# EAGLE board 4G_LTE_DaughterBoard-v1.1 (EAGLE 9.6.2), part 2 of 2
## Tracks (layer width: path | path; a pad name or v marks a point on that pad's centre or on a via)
$$$29
  Bottom 0.203: U11.8 R17.1
  Bottom 0.305: R17.1 R18.2
+BAT  (via drill 0.35)
  Top 0.508: U3.3 19.02,104.75 | 22.34,99.86 22.29,99.91 v22.32,99.94 | v18.14,103.86 18.24,103.96
  Top 0.61: 19.02,104.75 C26.1 18.24,103.96 | BATTERY.2 22.34,99.86
  Bottom 0.61: v22.32,99.94 20.94,99.94 18.14,102.74 v18.14,103.86
  pour Top (isolate 0.254, no thermals): 28.27,101.11 35.49,101.11 36.05,100.55 36.05,98.89 35.74,98.58 33.85,98.58 33.47,98.96 28.27,98.96
AGND  (via drill 0.3)
  Top 0.406: J3.2 36.16,114.78 v35.95,114.99
  Bottom 0.203: U7.7 41.78,105.72 41.96,105.54 41.96,104.75 42.38,104.33 42.38,103.64 42.43,103.59 42.43,102.87 C51.2 | U7.18 36.73,105.72 36.38,105.36 36.38,105.16 36.18,104.96 35.78,104.96 | C57.1 C56.1 | C56.1
  Bottom 0.305: v45.19,105.6 45.19,105.96 45.28,106.05 45.28,107.82 v45.1,108
  other vias: 44.92,102.31 34.37,105.21 34.67,103.11 30.45,110.39 25.85,107.69 40.75,101.89 40.85,98.49 44.25,98.69
  pour Bottom (isolate 0.254, rank 2, no thermals): 22.78,96.56 22.78,115.76 41.18,115.76 41.38,115.56 41.38,113.76 41.48,113.36 41.58,112.76 41.78,112.36 41.98,112.06 44.93,111.59 45.58,111.26 45.58,99.86 45.41,96.56
  pour Route2 (isolate 0.254): 22.78,115.76 22.78,96.56 45.38,96.56 45.38,111.46 45.08,111.76 43.38,111.76 41.48,113.66 41.48,115.76
ANT_DIV
  Top 0.293: U1.35 30.77,45.7 arc45 31.13,44.82 arc45 32.48,44.26 35.82,44.26 arc90 37.97,46.41 C70.2 38.98,56.62 L3.1
ANT_GNSS
  Top 0.293: U1.47 C74.2 38.97,62.59 C83.2
ANT_MAIN
  Top 0.293: U1.49 C68.2 38.97,68.29 L2.1
AP_READY_EC25  (via drill 0.3, 0.41)
  Top 0.203: U1.2 v2.34,73.5 v2.33,73.49
  Route2 0.203: v3.5,22.12 3.5,21.95 9.69,15.76 13.4,15.76 14.38,14.78 v14.38,12.46
  Bottom 0.203: Q6.3 14.28,11.66 R44.2 v14.38,12.46 | v2.33,73.49 3.04,73.49 5.97,70.56 5.97,61.5 5.15,60.67 5.15,52.04 6.78,50.41 6.78,43.19 2.22,38.63 2.22,23.79 3.48,22.53 3.48,22.14 v3.5,22.12
BT_EN  (via drill 0.3)
  Top 0.203: U1.139 6.52,53.09 v5.81,52.38 | v22,36.75 22,34.82 22.3,34.52 U2.10 27.35,34.52 C19.1
  Route2 0.203: v22,36.75 22,36.67 21.56,36.23 9.79,36.23 9.49,35.93 9.49,35.92 9.27,35.7 6.45,35.7 6.21,35.94 6.21,46.59 5.56,47.24 v5.56,47.87
  Route15 0.203: v5.81,52.38 5.81,47.93 5.75,47.87 v5.56,47.87
CODEC_PCM_CLK  (via drill 0.3)
  Top 0.203: R38.1 20.33,44.8 v20.33,42.67
  Route2 0.203: v42.68,89.48 42.68,88.43 39.79,85.54 39.79,79.12 37.21,76.54 32.73,76.54 28.85,72.66 28.85,55.45 23.48,50.08 23.48,45.09 21.06,42.67 v20.33,42.67
  Route15 0.203: v33.76,110.24 33.95,110.05 34.52,110.05 36.33,108.24 38.66,108.24 39.18,107.73 39.18,95.36 42.38,92.16 42.38,89.78 v42.68,89.48
  Bottom 0.152: v33.76,110.24 33.78,110.22 33.78,110.06
  Bottom 0.203: R66.2 34.57,110.06 33.78,110.06
CODEC_PCM_IN  (via drill 0.3)
  Top 0.203: R32.1 16.42,44.79 v16.42,42.9
  Route2 0.203: v41,91.46 40.4,90.86 40.4,87.67 38.72,85.99 38.72,79.56 36.77,77.61 32.28,77.61 27.78,73.1 27.78,55.89 22.41,50.52 22.41,45.58 21.04,44.21 17.73,44.21 v16.42,42.9
  Route15 0.203: v32.55,106.14 32.56,106.13 36.02,106.13 38.11,104.04 38.11,94.35 v41,91.46
  Bottom 0.203: R69.2 34.65,107.32 33.65,106.32 32.72,106.32 v32.55,106.14 C53.2
CODEC_PCM_OUT  (via drill 0.3)
  Top 0.203: R34.1 17.73,44.8 v17.73,42.67
  Route2 0.203: v41.24,90.08 40.9,89.74 40.9,87.66 39.08,85.84 39.08,79.41 36.92,77.25 32.43,77.25 28.14,72.96 28.14,55.74 22.77,50.38 22.77,45.39 21.22,43.84 19.04,43.84 17.87,42.67 v17.73,42.67
  Route15 0.203: v32.77,109.63 33.12,109.28 33.12,108.86 33.95,108.03 34.62,108.03 38.47,104.18 38.47,95.04 41.67,91.85 41.67,90.51 v41.24,90.08
  Bottom 0.203: R68.2 33.87,108.12 33.77,108.22 33.77,108.43 C54.2 32.77,109.43 v32.77,109.63
CODEC_PCM_SYNC  (via drill 0.3)
  Top 0.203: R36.1 19.08,42.9 v19.03,42.85
  Route2 0.203: v41.69,88.89 41.69,87.95 39.43,85.69 39.43,79.26 37.06,76.9 32.58,76.9 28.49,72.81 28.49,55.59 23.12,50.23 23.12,45.24 21.36,43.47 19.65,43.47 v19.03,42.85
  Route15 0.203: v41.69,88.89 41.69,89.6 42.02,89.94 42.02,92.01 38.83,95.21 38.83,104.43 v34.28,108.98
  Bottom 0.203: R67.2 34.78,108.98 v34.28,108.98
CODEC_POWER_EN  (via drill 0.3, 0.35)
  Top 0.203: v15.15,81.45 15.11,81.45 14.45,82.11 14.45,88.43 14.88,88.86 15.93,88.86 16.38,89.31 Q10.1 | v26.08,7.92 7.02,7.92 v2.13,12.81
  Route15 0.203: v15.15,81.45 15.15,75.62 14.48,74.95 14.48,74.41 16.12,72.77 29.05,72.77 32.77,69.05 32.77,57.19 31.94,56.37 31.94,49.08 32.95,48.07 32.95,37.3 35.29,34.96 35.29,22.07 28.09,14.87 28.09,10.02 26.08,8.01 v26.08,7.92
  Bottom 0.203: WIPHONE_DAUGHTERBOARD-FOOTPRINT1.17 2.48,12.46 v2.13,12.81
COEX_UART_RX  (via drill 0.3)
  Top 0.203: U1.137 6.52,57.01 v5.9,56.39 | v22.45,29.02 v22.47,29 22.49,29.02 U2.5 27.4,29.02 R29.1
  Route2 0.203: v2.68,41.02 4.55,39.15 4.55,29.62 5.18,29 7.34,29 8.27,29 10.06,27.22 20.66,27.22 v22.45,29.02
  Route15 0.203: v5.9,56.39 3.77,54.26 3.77,49.64 1.58,47.45 1.58,42.12 v2.68,41.02
COEX_UART_TX  (via drill 0.3)
  Top 0.203: U1.138 6.52,55.05 v5.9,54.43 | v22.25,30.01 24.01,30.01 U2.6 27.42,30.12 R28.1
  Route2 0.203: v3.53,41.56 4.91,40.18 4.91,29.77 5.33,29.35 7.19,29.35 7.2,29.36 8.42,29.36 10.2,27.57 19.84,27.57 22.2,29.93 22.2,30.01 v22.25,30.01
  Route15 0.203: v5.9,54.43 4.13,52.67 4.13,49.51 1.99,47.37 1.99,43.1 v3.53,41.56
CTS_BT  (via drill 0.3)
  Top 0.203: U1.40 v33.31,53.5 | U2.8 25.87,32.32 26.15,32.6 v26.49,32.6
  Route2 0.203: v33.31,53.5 33.31,53.41 24.32,44.43 v24.32,39.83
  Bottom 0.203: v24.32,39.83 25.3,38.85 25.3,33.59 26.29,32.6 v26.49,32.6
DBG_RXD
  Top 0.203: U1.11 TP1.P$1
DBG_TXD
  Top 0.203: U1.12 2.15,57.4 TP2.P$1
DBG_TXD_FC20
  Top 0.203: U2.4 26.35,27.92 27.26,27.92 R30.1
DTR  (via drill 0.35)
  Route2 0.203: v7.35,8.64 7.35,7.84 v6.65,7.14
  Bottom 0.203: R86.1 R85.1 7.42,7.14 v6.65,7.14 | WIPHONE_DAUGHTERBOARD-FOOTPRINT1.20 7.35,8.54 v7.35,8.64
FC20_ANT
  Top 0.293: L4.1 8.09,25.86 C72.2 11.24,25.86 U2.30
GND  (via drill 0.3, 0.35, 0.41, 0.5)
  Top 0.203: C18.2 28.88,32.99 v28.99,33.1
  Top 0.229: U1.19 9.97,49.32 10.21,49.56 13.65,49.56 13.87,49.34 U1.22
  Top 0.305: D3.A 37.27,102.33 C90.1 | R58.2 16.83,84.02 17.95,84.02 v18.37,84.44 | v22.43,13.84 22.26,13.67 16.47,13.67 16.28,13.86 | 15.98,14.16 v15.98,16.9 | 16.28,13.86 15.98,14.16 | v16.28,13 16.28,13.86 | 15.98,14.16 15.66,13.84 v9.23,13.84 9.23,17.59 v9.59,17.95
  Top 0.406: U3.2 18.34,106.06 v18.3,106.1
  Top 0.508: C45.1 C44.1 17.34,86.56 U5.2 v20.88,86.56 | Q10.2 17.38,88.79 v17.1,88.51
  Route2 0.203: v2.55,16.44 2.55,13.32 2.79,13.08 2.79,9.9 6.87,5.82 v8.49,5.82
  Route15 0.305: v35.98,14.06 35.98,13.16 37.88,11.26 37.88,8.56 37.68,8.36 v37.48,8.36
  Bottom 0.203: C65.1 C66.1 | C53.1 32.5,104.56 v31.89,104.56 v31.88,104.56 | C52.1 34.35,111.08 v34.35,111.49 | C54.1 31.64,108.82 v31.28,108.45 | C65.1 39.33,112.61 v39.48,112.76 | WIPHONE_DAUGHTERBOARD-FOOTPRINT1.13 3.43,17.32 v2.55,16.44 | v8.49,5.82 8.49,6.05 R86.2 | C67.1 C65.1 | K1.1 25.76,113.69 D6.2 26,113.93 C86.1 C85.1
  Bottom 0.293: C1.2 5.8,30.75 v5.68,30.63 | 11.23,14.06 10.58,14.06 C22.2 9.36,13.84 v9.23,13.84 | C21.2 15.53,14.56 15.9,14.19 16.28,13.81 v16.28,13 | D10.2 23.69,17.51 23.69,15.1 v22.43,13.84 | C20.2 15.38,17.96 | 4.66,18.73 7.58,18.73 8.35,17.95 v9.59,17.95
  Bottom 0.305: WIPHONE_DAUGHTERBOARD-FOOTPRINT1.2 42.81,18.81 37.24,18.81 36.25,17.82 36.25,17.08 35.98,16.82 | 4.66,18.73 4.62,18.73 WIPHONE_DAUGHTERBOARD-FOOTPRINT1.13 | 15.46,17.96 16.19,17.96 16.72,18.49 Q1.2 | 15.46,17.96 15.38,17.96 | v15.98,16.9 15.46,17.42 15.46,17.96 | R45.2 37.5,16.23 36.91,16.82 35.98,16.82 | D10.2 28.45,15.95 | U6.7 28.45,15.95 | v35.98,14.06 35.98,16.82 | 28.45,15.95 30.02,17.52 33.66,17.52 R52.1 34.36,16.82 35.98,16.82 | Q2.2 11.09,17.95 v9.59,17.95 | Q3.2 16.13,14.19 15.9,14.19 | 11.23,14.06 11.68,14.51 Q4.2 | C81.2 28.84,7.66 36.78,7.66 v37.48,8.36 36.3,9.54 C27.2
  Bottom 0.508: U7.33 38.42,106.72 v38.38,106.76 | U7.33 39.13,106.72 v38.38,105.96 | U7.33 39.22,106.72 v38.38,107.56 | 6.58,24.16 6.58,22.59 5.19,21.19 4.54,21.19 WIPHONE_DAUGHTERBOARD-FOOTPRINT1.11 WIPHONE_DAUGHTERBOARD-FOOTPRINT1.13 | 44.07,24.39 v43.91,24.56
  Bottom 1.016: WIPHONE_DAUGHTERBOARD-FOOTPRINT1.2 43.91,20.24 v43.91,24.56
  other vias: 19.9,92.52 9.42,109.38 21.38,89.76 17.49,105.88 28.47,103.45 21.36,84.45 19.32,115.45 21.87,113.54 21.9,115.37 19.02,114.49 9.75,112.05 8.58,112.16 8.17,110.92 9.3,110.85 15,115.3 37.5,69.62 38.37,69.59 39.23,69.59 40.09,69.55 40.99,69.55 41.85,69.55 37.47,66.29 38.33,66.25 39.19,66.25 40.05,66.21 40.95,66.21 41.82,66.21 38.82,55.14 39.68,55.14 40.44,55.2 41.24,55.2 42.1,55.2 5.99,24.65 6.85,24.65 7.72,24.65 8.62,24.65 9.48,24.65 41.18,63.62 37.72,63.66 38.58,63.66 39.44,63.62 40.34,63.62 37.43,60.59 38.29,60.55 39.15,60.55 40.02,60.51 40.92,60.51 41.78,60.51 37.43,57.85 38.29,57.81 39.15,57.81 40.02,57.77 40.92,57.77 41.78,57.77 15.48,86.23 30.52,87.62 27.08,88.3 27.16,89.73 27.31,91.09 10.3,85.77 10.32,88.65 10.11,91.67 8.75,90.46 7.74,86.23 8.48,81.53 4.93,81.28 7.35,79.61 14.88,97.74 15.05,100.33 22,96.72 26.55,93.39 27.97,44.41 30.36,42.02 37.64,24.62 28.33,24 38.51,32.53 36.76,32.53 35.85,84.21 36.77,80.7 13.61,45.89 25.91,23.86 21.71,25.26 19.51,25.16 17.11,25.16 14.71,25.16 40.31,24.66 27.91,53.16 20.61,69.44 19.41,69.44 17.21,69.46 11.41,71.86 21.01,71.36 24.61,71.16 9.91,74.36 36.01,88.96 36.41,92.76 42.61,84.06 31.01,91.56 4.91,101.06 8.31,99.26 2.49,101.02 2.49,97.22 2.41,61.26 2.51,62.66 16.13,109.12 16.11,108.28 12.01,109.94 11.81,112.22 18.71,112.32 11.85,108.9 19.17,108.36 20.21,108.28 21.95,110.66 21.99,109.82 18.31,69.46 15.45,67.3 15.45,66.3 15.43,64.1 15.43,65.2 15.45,62.8 15.45,61.8 15.43,59.6 15.43,60.7 19.45,68.3 19.45,67.1 19.43,66 22.75,68.5 22.75,67.5 22.73,66.4 25.81,69.24 24.61,69.44 21.81,69.46 23.31,69.46 26.25,68 26.25,67 26.23,64.8 26.23,65.9 26.25,63.5 26.25,62.5 26.23,60.3 26.23,61.4 26.25,59 26.25,58 26.23,55.8 26.23,56.9 25.01,54.74 24.01,54.74 21.81,54.76 22.91,54.76 20.01,54.74 19.01,54.74 16.81,54.76 17.91,54.76 16.25,58.5 16.25,57.5 16.23,55.3 16.23,56.4 17.19,58.84 18.19,58.84 20.39,58.83 19.29,58.83 21.69,58.84 22.69,58.84 25.09,59.63 23.99,59.63 16.23,65.8 23.65,62.8 23.65,61.8 23.63,60.7 25.01,64.54 23.71,64.56 22.95,57.8 22.95,56.8 22.93,55.7 19.55,58 19.55,57 19.53,55.9 22.75,54 22.75,53 22.75,51.99 19.55,53.6 19.55,52.6 19.53,51.5 16.15,53.6 16.15,52.6 16.13,51.5 21.01,50.24 20.01,50.24 17.81,50.26 18.91,50.26 28.75,54.2 28.75,53.2 28.73,52.1 19.35,71.6 19.35,70.6 12.93,72.95 12.9,71.88 12.9,70.79 10.96,74.19 12.08,74.14 13.24,74.16 26.87,69.25 16.84,50.28 26.33,51.46 30.63,67.56 30.63,66.27 30.63,65.02 30.63,63.75 30.63,62.48 30.62,61.39 30.61,60.43 4.46,77.32 5.59,77.29 5.6,76.14 4.38,76.14 5.83,74.99 6.96,74.46 8.2,74.43 9.8,73.39 16.13,28.47 17.33,28.47 18.51,28.46 19.58,28.51 19.63,29.65 19.61,30.76 19.59,31.88 19.6,32.98 15.88,33.38 17.01,33.4 18.09,33.4 15.88,31.8 15.98,30.75 15.99,29.62 16.97,32.22 17.05,31.18 17.11,29.59 18.27,29.52 18.55,30.61 18.47,31.7 18.67,32.59 36.81,26.86 36.81,25.62 37.96,26.81 38.02,25.64 39.21,25.6 40.49,25.6 41.79,25.69 43.01,25.62 44.35,25.6 43.72,26.84 43.77,28.09 43.83,29.31 43.88,30.48 44,31.64 44,32.82 44.01,34.18 43.96,35.41 43.95,36.75 42.7,36.84 41.2,36.77 40.05,37.72 39.01,38.53 38.18,39.26 38.51,40.4 38.37,41.68 38.34,42.99 38.47,44.19 38.75,45.09 38.97,45.91 39.12,46.83 39.21,47.75 39.21,48.62 39.22,49.5 39.27,50.42 39.23,51.27 39.18,52.13 39.21,53.08 37.79,71.21 37.83,72.48 37.82,73.71 37.82,74.83 39.09,75.6 40.35,76.68 41.24,77.55 41.79,79.11 42.02,80.52 42.02,82.33 42.05,85.03 43.45,85.78 39.39,71.21 39.64,72.54 39.53,73.77 40.68,74.98 41.07,73.2 41.22,71.5 31.35,92.8 32.87,93.14 32.54,91.55 34.8,90.08 28.33,93.57 24.89,93.57 23.39,93.87
  pour Top (isolate 0.203, rank 3): -0.02,3.76 -0.02,113.36 arc-90 4.08,117.46 43.78,117.46 arc-90 47.48,113.76 47.48,3.46 arc-90 43.98,-0.04 3.78,-0.04 arc-90
  pour Bottom (isolate 0.305, rank 3): -0.12,3.86 -0.12,113.46 arc-90 3.98,117.56 43.68,117.56 arc-90 47.38,113.86 47.38,3.56 arc-90 43.88,0.06 3.68,0.06 arc-90
  pour Route2 (isolate 0.305, rank 2, no thermals): -0.02,3.76 -0.02,113.26 arc-90 4.18,117.46 43.88,117.46 arc-90 47.48,113.86 47.48,3.76 arc-90 43.68,-0.04 3.78,-0.04 arc-90
  pour Route15 (isolate 0.381): -0.01,93.19 -0.01,112.78 0,112.79 0,113.67 arc-90 3.83,117.5 43.82,117.5 arc-90 47.51,113.81 47.51,7.55 47.52,7.54 47.52,3.96 arc-90 43.54,-0.02 3.95,-0.02 arc-90 0,3.93 0,93.13
  pour Top (no thermals): 10.15,50.54 10.15,73.54 10.35,73.74 29.15,73.74 29.35,73.54 29.75,73.14 29.75,51.34 29.55,51.14 28.95,50.54
I2C_SCL  (via drill 0.3)
  Top 0.203: U1.41 v33.61,54.8
  Route2 0.203: v33.61,54.8 29.2,59.21 29.2,72.47 32.92,76.19 37.36,76.19 40.14,78.97 40.14,85.4 42.53,87.79 43.38,87.79 v44.1,88.51
  Route15 0.203: v35.66,111.44 36.39,110.72 37.75,110.72 39.9,108.58 39.9,95.65 43.09,92.45 43.09,90.5 43.69,89.9 43.69,88.98 44.1,88.57 v44.1,88.51
  Bottom 0.203: U7.26 38.33,109.19 38.09,109.43 37.78,109.43 37.75,109.4 37.21,109.4 36.43,110.18 36.43,111.44 36.42,111.45 R64.1 36.42,111.61 36.34,111.53 36.26,111.44 v35.66,111.44
I2C_SDA  (via drill 0.3)
  Top 0.203: U1.42 v33.61,56.1
  Route2 0.203: v33.61,56.1 29.56,60.15 29.56,72.32 33.07,75.83 37.51,75.83 40.5,78.82 40.5,85.25 42.42,87.17 v44.48,87.17
  Route15 0.203: v37.48,110.06 39.54,108 39.54,103.95 39.54,95.5 42.73,92.31 42.73,90.35 43.33,89.75 43.33,87.96 44.12,87.17 v44.48,87.17
  Bottom 0.203: U7.27 38.73,109.29 37.96,110.06 v37.48,110.06 37.33,110.21 R63.1
L/EARPIECE  (via drill 0.3)
  Top 0.152: C89.2
  Top 0.203: C89.2 C90.2 36.27,102.79 D3.C 36.06,102.03 35.65,102.44 35.65,103.5 35.22,103.93 32.42,103.93 v32.06,103.57 | J3.4 35.23,106.3 35.23,104.74 C89.2
  Bottom 0.203: C48.2 33.33,104.48 32.81,103.96 32.28,103.96 32.06,103.74 v32.06,103.57
MIC+  (via drill 0.3, 0.35)
  Top 0.152: v31.71,112.67 31.85,112.81 36.38,112.81 38.45,110.73 40.34,110.73 42,109.07 42,107.96 42.37,107.59 43.19,107.59 v43.28,107.5
  Route15 0.152: v31.71,112.67 26.79,112.67 26.13,113.33 25.16,113.33 25.15,113.34 25,113.19 v24.7,113.19
  Bottom 0.152: U7.3 41.83,107.32 42.18,107.66 43.13,107.66 v43.28,107.5 | v24.7,113.19 24.95,113.44 C76.2
MIC-  (via drill 0.3, 0.35)
  Top 0.152: v31.89,111.68 31.96,111.68 32.7,112.43 36.33,112.43 38.33,110.43 40.06,110.43 41.7,108.79 41.7,107.74 v42.48,106.96
  Route15 0.152: v31.89,111.68 26.24,111.68 26.13,111.57 25.4,111.57 24.82,112.14 v24.35,112.14
  Bottom 0.152: U7.4 42.43,106.92 v42.48,106.96 | v24.35,112.14 24.95,111.54 C77.2
MIC_N
  Bottom 0.152: R76.1 24.2,110.27 C77.1 25.45,110.77 25.45,110.94 25.95,111.44 26.25,111.44 26.55,111.74 26.55,112.04 27.03,112.52 27.12,112.52 27.12,112.44
  Bottom 0.203: C80.2 C79.2 27.12,112.52
MIC_P  (via drill 0.35)
  Top 0.203: 28.98,114.33 J3.1 28.62,115.14 v28.05,115.14
  Bottom 0.203: C86.2 26.87,114.93 | R75.2 C76.1 25.03,114.92 D6.1 26.7,114.92 C86.2 | C86.2 C85.2 27.75,114.84 v28.05,115.14
MICBIAS  (via drill 0.35)
  Top 0.203: v44.97,109.65 44.51,109.65 44.29,109.43 42.9,109.43 40.73,111.6 38.86,111.6 36.79,113.67 31.21,113.67 v31.19,113.69
  Route15 0.203: v31.19,113.69 30.79,114.09 24.84,114.09 23.48,115.45 v23.2,115.45
  Bottom 0.203: v44.97,109.65 44.97,109.57 C55.1 44.62,109.28 R70.1 | v23.2,115.45 23.39,115.26 R60.1
N$1
  Bottom 0.203: U7.14 38.73,103.77 C4.1
N$2
  Bottom 0.203: U7.13 39.13,103.37 C4.2
N$3
  Bottom 0.203: U7.12 39.53,103.86 C8.1
N$4
  Top 0.203: U2.32 14.39,22.45 14.39,20.96 14.11,20.68 10.23,20.68 R1.2
N$5  (via drill 0.3)
  Top 0.152: 10.03,29.02 v10.01,29.04
  Top 0.293: U2.27 10.03,29.02
  Bottom 0.293: R24.1 8.16,27.79 R3.2 9.49,28.52 v10.01,29.04
N$6  (via drill 0.3)
  Top 0.152: v9.97,30.08 v9.97,30.07
  Top 0.293: U2.26 11.34,30.08 v9.97,30.08
  Bottom 0.152: 9.92,30.02 v9.97,30.07
  Bottom 0.293: R23.1 9.92,30.02
  Bottom 0.305: R23.1 | R23.1 R4.2 | C1.1 R23.1
N$7  (via drill 0.3)
  Top 0.293: U2.25 10.04,31.22 v9.99,31.26
  Bottom 0.152: R22.1 8.17,31.49
  Bottom 0.293: 8.17,31.49 R5.2 9.77,31.48 v9.99,31.26
N$8  (via drill 0.3)
  Top 0.203: v9.94,32.31 v9.95,32.32
  Top 0.293: v9.95,32.32 U2.24
  Bottom 0.293: R21.1 8.18,33.6 R12.2
  Bottom 0.305: R12.2 9.34,32.91 v9.94,32.31
N$9  (via drill 0.3)
  Top 0.293: U2.23 11.36,33.4 v9.94,33.4
  Bottom 0.293: R20.1 8.18,34.33 R13.2 9.02,34.32 v9.94,33.4
N$10  (via drill 0.3)
  Top 0.293: U2.22 9.98,34.52 v9.97,34.53
  Bottom 0.152: R14.2 R19.1
  Bottom 0.293: R14.2 | R19.1 8.75,35.75 v9.97,34.53
N$11
  Top 0.203: U2.19 14.45,40.89 R25.2 13.6,40.9 C17.2
N$12  (via drill 0.3, 0.35)
  Top 0.305: U1.24 v16.47,46.29 16.47,45.77 R32.2
  Route15 0.203: v16.47,46.29 18.89,43.87 23.83,43.87 30.46,37.23 30.46,36.26 32.66,34.07 32.66,24.24 24.51,16.1 v24.51,15.53
  Bottom 0.152: R31.2 24.51,15.37 v24.51,15.53
N$13
  Bottom 0.203: U11.1 39.29,33.75 R46.1
N$14  (via drill 0.3, 0.35)
  Top 0.203: 17.73,45.81 R34.2 | 17.77,46.42 v17.77,46.27
  Top 0.305: U1.25 17.77,46.42 | v17.77,46.27 17.77,45.85 17.73,45.81
  Route15 0.203: v17.77,46.27 19.82,44.22 23.97,44.22 30.82,37.38 30.82,36.41 33.01,34.22 33.01,24.09 25.29,16.37 25.29,13.43 24.88,13.02 v24.08,13.02
  Bottom 0.203: R33.2 24.94,12.16 v24.08,13.02
N$15  (via drill 0.3)
  Top 0.203: U1.67 v16.47,74.79 v16.46,74.78
  Route15 0.203: v16.46,74.78 17.58,73.66 29.38,73.66 33.69,69.35 33.69,57.11 32.65,56.07 32.65,49.43 33.67,48.41 33.67,37.59 36,35.25 36,18.47 v36.95,17.52 v36.95,17.53
  Bottom 0.203: v36.95,17.53 37.97,17.53 R41.2
N$16  (via drill 0.3, 0.35)
  Top 0.203: 19.03,45.81 R36.2 | 19.07,46.37 v19.07,46.21
  Top 0.305: U1.26 19.07,46.37 | v19.07,46.21 19.07,45.85 19.03,45.81
  Route15 0.203: v19.07,46.21 20.7,44.58 24.12,44.58 31.18,37.52 31.18,36.56 33.37,34.37 33.37,23.8 25.78,16.21 25.78,13.21 24.58,12.01 v23.78,12.01
  Bottom 0.203: R35.2 24.38,12.01 v23.78,12.01
N$17  (via drill 0.3)
  Top 0.203: 15.22,76.4 15.22,74.76 v15.14,74.68
  Top 0.305: U1.68 15.22,76.4
  Route15 0.203: v15.14,74.68 16.7,73.12 29.25,73.12 33.12,69.25 33.12,57.05 32.3,56.22 32.3,49.29 33.31,48.27 33.31,37.44 35.65,35.11 35.65,16.93 v37.11,15.47
  Bottom 0.203: R42.2 37.17,15.41 v37.11,15.47
N$18  (via drill 0.3, 0.35)
  Top 0.203: 20.37,46.42 v20.37,46.24 | R38.2 20.28,45.95 20.37,46.04
  Top 0.305: U1.27 20.37,46.42 | v20.37,46.24 20.37,46.04
  Route15 0.203: v20.37,46.24 21.67,44.93 24.27,44.93 31.53,37.67 31.53,36.71 33.72,34.51 33.72,23.51 26.81,16.6 26.8,16.6 26.28,16.07 26.28,13.06 24.2,10.98 24.19,10.99 v24.09,10.99
  Bottom 0.203: R37.2 24.82,10.46 24.29,10.99 v24.09,10.99
N$19
  Bottom 0.305: R82.2 21.11,20.27 R81.1
N$20  (via drill 0.3)
  Top 0.305: R11.1 2.12,92.96 2.15,92.99 v2.1,93.04 | D8.C 6.24,99.02 v6.39,98.86
  Route15 0.305: v2.1,93.04 6.37,97.3 6.37,98.86 v6.39,98.86
N$21
  Top 0.229: U1.69 13.87,78.59 FL1.3
N$22
  Bottom 0.203: R46.2 C24.2
N$23
  Top 0.305: R50.2 10.27,99.87 9.13,101.02 D2.C
N$24  (via drill 0.3)
  Top 0.305: R50.1 11.19,100.45 v11.1,100.54 | v17.91,107.24 19.15,107.24 U3.1
  Route15 0.305: v17.91,107.24 17.91,107.15 17.47,107.15 16.32,106 16.32,104.81 13.83,102.32 12.88,102.32 v11.1,100.54
N$25
  Top 0.152: U3.5 22.08,107.11 R51.2
N$26
  Top 0.229: U1.70 12.57,78.66 FL1.4
N$27
  Top 0.305: R11.2 3.03,91.47 3.46,91.04 Q11.3
N$28
  Bottom 0.203: U11.7 R16.1
N$29
  Bottom 0.203: Q6.1 13.23,9.26 C23.2 R43.2
N$30
  pour Bottom (isolate 0.254, no thermals): 32.71,31.38 28.98,31.38 28.89,31.29 28.89,27.78 29,27.67 32.85,27.67 32.85,31.27 32.75,31.37
N$31
  Top 0.305: U4.4 22.57,91.51 R53.2 R54.1
N$32
  Top 0.203: U4.3 17.43,91.51 16.88,90.96 Q10.3
  Top 0.305: R55.1 18.88,91.46 U4.3
N$33
  Top 0.203: U5.4 22.03,86.72 R57.1 R56.2
N$34
  Top 0.152: U5.3 18.03,85.61 17.88,85.46 R59.2 17.14,84.7 R58.1
N$35  (via drill 0.3)
  Top 0.203: R8.1 29.63,84.46 D5.4 29.69,83.69 31.94,81.44 J1.C7 v34.2,81.45
  Bottom 0.203: v34.2,81.45 34.18,81.47 34.29,81.58 R9.2 35.06,82.31 C5.1
N$36  (via drill 0.3)
  Top 0.203: v31.75,82.81 31.24,82.81 30.34,83.71 D5.5 30.34,85.23 30.2,85.37 27.48,85.37 27.39,85.29 R7.1 | J1.C3 32.42,80.17 v31.96,80.63
  Route15 0.203: v31.75,82.81 31.96,82.6 v31.96,80.63
  Bottom 0.203: C6.1 32.1,80.49 v31.96,80.63
N$37  (via drill 0.3)
  Top 0.203: D5.6 31.15,84.52 v31.76,83.91 32.96,82.71 J1.C2 | 28.23,83.73 v28.29,83.67
  Top 0.229: R6.1 27.44,83.73 28.23,83.73
  Route2 0.203: v28.29,83.67 28.53,83.91 v31.76,83.91
  Bottom 0.203: C7.1 32.49,83.18 v31.76,83.91
N$38
  Bottom 0.203: U7.11 39.93,104.14 40.24,103.82 40.48,103.82 C8.2
N$39
  Bottom 0.203: U7.17 36.43,104.42 R61.2
N$40
  Bottom 0.203: U7.20 R62.2
N$41
  Bottom 0.203: C47.1 33.78,103.85 34.35,104.42 R61.1
N$42
  Bottom 0.203: R62.1 34.67,106.52 33.67,105.52 C48.1
N$43
  Bottom 0.203: U7.16 37.52,104.71 36.42,103.62 C49.1
N$44
  Bottom 0.203: U7.19 36.21,106.12 35.81,105.72 C50.1
N$45
  Bottom 0.203: C51.1 41.33,103.87 U7.8
N$46
  Bottom 0.203: R65.1 42.46,108.12 U7.1
N$47
  Bottom 0.203: U7.22 36.79,107.32 36.34,107.76 35.99,108.12 R68.1
N$48
  Bottom 0.203: U7.21 36.62,106.92 36.22,107.32 R69.1
N$49
  Bottom 0.203: U7.24 36.83,108.62 36.83,109.1 36.11,109.81 R66.1 C52.2
N$50
  Bottom 0.203: U7.23 36.89,107.72 36.7,107.91 36.7,108.1 35.78,109.02 R67.1
N$51
  Bottom 0.152: R70.2 42.78,109.26 42.24,108.72 U7.32
N$52
  Bottom 0.203: U7.15 38.33,104.04 38.14,103.85 37.56,103.85 37.43,103.72 C64.2 C63.2 C62.2 35.54,102.77 R74.2
N$53
  Bottom 0.203: R71.2 C58.2 43.09,105.42 41.99,106.52 U7.5
N$54
  Bottom 0.203: U7.6 41.89,106.12 42.96,105.04 42.96,104.3 43.47,103.79 C57.2 C56.2 | C56.2 43.47,102.11 R72.2 | C56.2
N$55
  Bottom 0.203: C67.2 40.13,109.75 39.93,109.55 U7.30
N$56
  Bottom 0.203: 40.92,110.04 41.3,109.67 42.34,109.67 R73.2 | 40.92,110.04 C59.2 | C61.2 C60.2 C59.2 | C59.2 40.92,110.04 | 40.92,110.04 40.33,109.45 U7.31
N$57
  Top 0.293: L3.2 40.95,56.64 arc-45 C71.2 42.53,56.61 arc90 ANT2.FEED
N$58
  Top 0.293: ANT3.FEED 5.28,25.89 C73.2 7.12,25.89 L4.2
N$59
  Top 0.293: C83.1 C75.2 41.44,62.63 42.14,62.63 | 42.14,62.63 42.44,62.63 | ANT4.FEED 42.14,62.63
N$60
  Bottom 0.203: 24.21,111.19 R76.2 24.18,111.19 R77.1 C78.1
N$61
  Top 0.293: ANT1.FEED 41.02,68.34 C69.2 40.93,68.34 L2.2
N$62
  Top 0.305: R78.2 6.85,92.45 Q12.3
N$63
  Top 0.305: R78.1 7.69,93.75 6.43,95.02 D9.C
N$64
  Bottom 0.203: R60.2 R75.1 23.37,113.13 C78.2
N$65
  Top 0.305: R39.1 10.19,95.95 9.13,97.02 D11.C
N$66  (via drill 0.35)
  Top 0.152: U1.62 22.97,74.67 v22.98,74.66
  Route2 0.203: v23.05,9.4 22.61,8.96 22.61,7.1 21.85,6.34 v19.85,6.34
  Route15 0.203: v26.1,71.73 29.09,71.73 32.06,68.76 32.06,57.49 31.23,56.66 31.23,48.79 32.24,47.77 32.24,37 34.57,34.68 34.57,22.55 27.15,15.13 27.15,10.49 25.93,9.26 23.18,9.26 v23.05,9.4
  Bottom 0.152: v22.98,74.66 25.68,71.96 25.98,71.96 26.1,71.84 v26.1,71.73
  Bottom 0.203: v19.85,6.34 9.56,6.34 R84.2
N$67
  Top 0.305: D7.C 5.89,103.91 R79.1
N$68
  cutout Route2 (isolate 0.254): 0.18,23.06 47.08,23.06 47.08,21.76 46.98,21.76 46.98,2.76 44.58,0.36 3.48,0.36 0.28,3.56 0.28,22.96
  cutout Route15 (isolate 0.254): 0.18,23.06 47.08,23.06 47.08,21.76 46.98,21.76 46.98,2.76 44.58,0.36 3.48,0.36 0.28,3.56 0.28,22.96
N$69
  Top 0.203: J1.CD 33.27,88.6 R47.2 33.18,88.69 30.04,88.69 29.69,88.34 D5.3 27.62,86.37 27.39,86.14 R48.1
N$70
  cutout Top (isolate 0.254): 0.18,23.06 0.18,3.56 3.38,0.36 44.58,0.36 46.98,2.76 46.98,23.06
  cutout Bottom (isolate 0.254): 0.28,23.06 0.28,3.56 3.48,0.36 44.68,0.36 47.08,2.76 47.08,23.06
N$71  (via drill 0.35)
  Top 0.203: U1.66 17.77,75.2 v17.44,74.88
  Route2 0.203: v22.96,10.65 22.26,9.95 22.26,7.25 22.15,7.14 v21.65,7.14
  Route15 0.203: v26.1,70.46 29.58,70.46 31.7,68.34 31.7,57.64 30.87,56.81 30.87,48.64 31.89,47.63 31.89,36.85 34.08,34.66 34.08,22.56 26.75,15.23 26.75,10.84 25.65,9.74 23.87,9.74 v22.96,10.65
  Bottom 0.203: v17.44,74.88 20.25,72.07 20.25,71.04 20.93,70.36 26.08,70.36 26.1,70.38 v26.1,70.46 | R85.2 7.53,5.56 7.95,5.14 9.65,5.14 10.15,5.64 20.75,5.64 21.65,6.54 v21.65,7.14
N$73
  Bottom 0.203: R89.1 R91.1 39.89,12.46 WIPHONE_DAUGHTERBOARD-FOOTPRINT1.7
N$74
  Bottom 0.203: R92.1 R90.1 39.59,9.92 WIPHONE_DAUGHTERBOARD-FOOTPRINT1.9
NET_MODE  (via drill 0.3)
  Top 0.203: v3.19,85.5 3.27,85.57 3.27,88.18 3.18,88.27 2.96,88.49 Q11.1 | U1.5 v2.44,69.6
  Route15 0.203: v2.44,69.6 2.44,70.12 2.99,70.67 2.99,82.13 2.05,83.07 2.05,84.34 3.25,85.54 3.24,85.54 v3.19,85.5
NET_STATUS  (via drill 0.3)
  Top 0.203: U1.6 2.39,68.3 v2.35,68.34
  Top 0.305: v5.9,87.18 5.9,88.93 6.35,89.38 Q12.1
  Route15 0.203: v2.35,68.34 3.34,69.34 3.34,82.28 2.45,83.17 2.45,84.24 2.95,84.74 3.75,84.74 5.9,86.89 v5.9,87.18
ON/OFF_MCU
  Bottom 0.203: WIPHONE_DAUGHTERBOARD-FOOTPRINT1.19 3.43,8.71 4.18,7.96 17.48,7.96 18.88,9.36 18.88,17.36 Q1.1
PCM_EN
  Bottom 0.305: U6.8 33.9,14.76 R52.2
PCMCLK_1.8V
  Bottom 0.152: R37.1 26.68,10.46 27.44,11.22 U6.2
PCMCLK_3.3V
  Bottom 0.203: U6.13 34.94,11.22 35.04,11.33 36.55,11.33 36.9,11.33 R90.2
PCMIN_1.8V
  Bottom 0.152: U6.5 26.74,13.16 R26.1 R31.1
  Bottom 0.203: 26.04,14.82 R31.1
PCMIN_3.3V
  Bottom 0.203: U6.10 36.18,13.17 37.15,14.14 R89.2
PCMOUT_1.8V
  Bottom 0.152: U6.4 27.34,12.52 26.98,12.16 R33.1 R83.1
PCMOUT_3.3V
  Bottom 0.203: U6.11 39.32,12.52 40.58,11.26 42.98,11.26 44.07,12.35 WIPHONE_DAUGHTERBOARD-FOOTPRINT1.8
PCMSYNC_1.8V
  Bottom 0.152: U6.3 27.39,11.87 26.78,11.26 R35.1
PCMSYNC_3.3V  (via drill 0.35)
  Route15 0.203: v40.08,10.76 42.58,8.26 v44.18,8.26
  Bottom 0.203: U6.12 38.87,11.87 39.98,10.76 v40.08,10.76 | v44.18,8.26 44.07,8.37 WIPHONE_DAUGHTERBOARD-FOOTPRINT1.10
PM_ENABLE  (via drill 0.3)
  Top 0.203: U1.127 9.7,52.02 9.7,50.45 10.06,50.09 15.35,50.09 15.48,50.22 v15.5,50.22
  Route2 0.203: v31.36,25.39 37.18,31.21 v38.65,31.21
  Route15 0.203: v15.5,50.22 15.81,49.91 15.81,46.02 16.19,45.63 16.6,45.63 18.72,43.51 23.68,43.51 30.11,37.08 30.11,36.12 32.3,33.92 32.3,26.33 v31.36,25.39
  Bottom 0.203: U11.3 v38.65,31.21 39.29,31.21 R15.1
PWRKEY  (via drill 0.3, 0.35)
  Top 0.203: U1.21 12.57,44.92 12.87,44.62 v13.66,44.62 | 23.5,110.14 23.5,110.33 21.38,112.45 K1.2 | 23.5,110.14 23.5,105.2 22.78,104.48 22.22,104.48 20.2,102.46 20.2,99.7 14,93.5 14,80.99 14.45,80.54 v14.45,80.32 | D14.1 23.5,110.14
  Route15 0.203: v13.66,44.62 14.01,44.62 15.37,43.26 15.37,43.02 16.38,42.01 21.07,42.01 24.36,38.72 27.44,38.72 29.4,36.76 29.4,35.82 31.59,33.63 31.59,27.73 30.69,26.83 30.69,22.95 26.28,18.54 19.32,18.54 | v14.45,80.32 14.45,75.42 14.13,75.1 14.13,74.26 15.98,72.41 28.91,72.41 32.41,68.9 32.41,57.34 31.58,56.51 31.58,48.93 32.6,47.92 32.6,37.15 34.94,34.81 34.94,22.31 27.54,14.91 27.54,10.37 25.47,8.31 22.73,8.31 20.28,10.76 20.28,12.07 19.32,13.03 19.32,18.54 | 19.32,18.54 v18.22,19.64
  Bottom 0.203: C20.1 15.65,19.38 16.42,20.14 17.72,20.14 v18.22,19.64 17.29,19.64 Q1.3
R/EARPIECE  (via drill 0.3)
  Top 0.203: C87.2 C88.2 25.42,105.56 D22.C | C87.2 26.88,105.86 27.74,106.72 27.74,107.05 29.16,108.47 29.16,109.24 29.16,111.24 | 29.16,111.49 29.16,111.24 | C87.2 v27.44,105.57 30.26,102.75 v32.6,102.75 | J3.3 29.16,111.24
  Bottom 0.152: C47.2 32.98,103.31
  Bottom 0.203: 32.98,103.31 32.6,102.93 v32.6,102.75
RESET_MCU
  Bottom 0.203: WIPHONE_DAUGHTERBOARD-FOOTPRINT1.15 3.43,15.21 4.38,16.16 8.18,16.16 8.98,16.96 12.03,16.96 12.48,17.41 Q2.1
RESET_N  (via drill 0.3, 0.35)
  Top 0.203: U1.20 11.27,45.17 12.78,43.66 v13.55,43.66
  Route2 0.203: v11.01,19.96 17.57,19.96 17.94,20.32 26.92,20.32 v27.01,20.23
  Route15 0.203: v13.55,43.66 14.47,43.66 15.02,43.11 15.02,42.82 16.2,41.64 20.94,41.64 24.21,38.37 27.29,38.37 29.04,36.61 29.04,35.68 31.23,33.48 31.23,27.88 30.33,26.97 30.33,23.41 27.15,20.23 v27.01,20.23
  Bottom 0.305: Q2.3 11.58,19.39 v11.01,19.96
RI  (via drill 0.35)
  Route2 0.203: v6.25,13.92 6.25,10.74 9.85,7.14 v10.35,7.14
  Bottom 0.203: WIPHONE_DAUGHTERBOARD-FOOTPRINT1.16 5.97,14.2 v6.25,13.92 | v10.35,7.14 10.24,7.03 R84.1
RTS_BT  (via drill 0.3)
  Top 0.203: U2.7 26.75,31.22 27.25,31.22 27.42,31.22 R27.1 27.36,31.28 v27.36,32.12 | U1.37 v33.42,49.6 v33.41,49.6
  Route2 0.203: v33.41,49.6 30.05,49.6 24.91,44.46 24.91,40.77 v25.11,40.57
  Bottom 0.203: v27.36,32.12 27.15,32.33 27.15,32.87 25.66,34.37 25.66,39 25.11,39.54 v25.11,40.57
RXD_BT  (via drill 0.3)
  Top 0.203: U2.17 16.57,38.91 v16.57,40.88 | U1.39 v29.87,52.19
  Route2 0.203: v16.57,40.88 17.35,41.66 21.05,41.66 24.19,44.8 24.19,47.28 27.88,50.97 29.05,50.97 29.87,51.79 v29.87,52.19
RXD_EC25
  Bottom 0.203: R45.1 42.75,16.23 WIPHONE_DAUGHTERBOARD-FOOTPRINT1.4
  Bottom 0.305: R42.1 R45.1
SDIO_CLK  (via drill 0.3)
  Top 0.152: 7.21,64.51 v7.21,64.46
  Top 0.293: U1.133 7.21,64.51
  Bottom 0.152: 6.79,29.26 6.77,29.24
  Bottom 0.293: v7.21,64.46 8.46,63.21 8.46,42.36 3.6,37.5 3.6,31.49 5.84,29.24 6.77,29.24 | R4.1 6.79,29.26
SDIO_CMD  (via drill 0.3)
  Top 0.152: 7.11,62.61 v7.11,62.53
  Top 0.293: U1.134 7.11,62.61
  Bottom 0.152: 6.85,28.52 6.78,28.6
  Bottom 0.293: v7.11,62.53 7.82,61.82 7.82,42.59 2.98,37.75 2.98,29.45 3.83,28.6 6.78,28.6 | R3.1 6.85,28.52
SDIO_D0  (via drill 0.3)
  Top 0.293: U1.132 v7.26,66.46
  Bottom 0.293: R5.1 5.29,31.48 4.26,32.52 4.26,37.25 9.06,42.06 9.06,64.65 v7.26,66.46
SDIO_D1  (via drill 0.3)
  Top 0.152: 7.23,68.49 v7.23,68.46
  Top 0.293: U1.131 7.23,68.49
  Bottom 0.293: R12.1 5.45,32.91 4.88,33.48 4.88,37.03 9.69,41.84 9.69,66 v7.23,68.46
SDIO_D2  (via drill 0.3)
  Top 0.293: U1.130 v7.26,70.46
  Bottom 0.293: v7.26,70.46 10.32,67.4 10.32,41.6 5.51,36.8 5.51,34.71 5.9,34.32 6.55,34.32 R13.1
SDIO_D3  (via drill 0.3)
  Top 0.293: U1.129 v7.26,72.46
  Bottom 0.293: v7.26,72.46 10.94,68.78 10.94,41.35 7.26,37.67 R14.1
SLEEP_STATUS
  Bottom 0.203: WIPHONE_DAUGHTERBOARD-FOOTPRINT1.18 8.87,9.56 Q6.2
STATUS  (via drill 0.3)
  Top 0.305: U1.61 24.27,74.75 v24.31,74.71 | v8.78,105 8.76,105 | 8.76,105 R79.2 | R49.2 8.1,105.66 8.76,105
  Route15 0.305: v24.31,74.71 20.74,78.28 20.74,84.07 19.19,85.62 19.19,100.58 16.14,103.63 v16.16,103.65
  Bottom 0.305: v16.16,103.65 11.48,103.65 10.13,105 v8.78,105
TXD_BT  (via drill 0.3)
  Top 0.203: U2.18 15.55,40.86 v15.57,40.88 | v24.74,50.41 32.66,50.41 33.16,50.9 U1.38
  Route2 0.203: v15.57,40.88 16.7,42.01 20.9,42.01 23.84,44.95 23.84,49.7 24.64,50.5 v24.74,50.41
TXD_EC25
  Bottom 0.203: R41.1 41.48,17.49 WIPHONE_DAUGHTERBOARD-FOOTPRINT1.3
USB_BOOT  (via drill 0.3)
  Top 0.203: U1.115 8.67,45.73 10.19,44.21 11.62,44.21 13.05,42.78 v12.93,42.66
  Route15 0.203: v12.93,42.66 12.93,42.6 12.93,42.59 15.3,40.22 16.84,40.22 17.8,41.18 20.89,41.18 24.07,38.01 27.01,38.01 28.69,36.33 28.69,35.53 30.88,33.34 30.88,28.03 29.97,27.12 29.97,23.81 27.51,21.34 v25.91,21.34
  Bottom 0.203: D10.1 25.91,20.83 v25.91,21.34
  Bottom 0.305: D10.1 25.23,20.27 R81.2
USB_N  (via drill 0.35)
  Top 0.261: FL1.1 12.95,80.29 12.95,106.51 13.56,107.12 v13.56,107.42 | 15.68,113.13 15.61,113.2 | 15.61,113.2 15.61,111.06 | 15.61,111.06 15.61,110.35 14.41,109.16 13.76,109.16 v13.46,108.86 | D4.C 15.61,111.06 | J2.2 15.61,113.2
  Bottom 0.261: v13.56,107.42 13.76,107.22 14.6,107.22 14.76,107.38 14.76,109.02 14.62,109.16 13.76,109.16 v13.46,108.86
USB_P  (via drill 0.35)
  Top 0.261: FL1.2 13.42,80.29 13.42,106.18 13.6,106.36 v13.9,106.36 | J2.3 14.95,111.04 | 14.95,111.04 14.95,110.35 14.22,109.62 13.76,109.62 v13.46,109.92 | D12.C 14.93,111.06 14.95,111.04
  Bottom 0.261: v13.9,106.36 13.9,106.56 14.1,106.76 14.79,106.76 15.22,107.19 15.22,109.21 14.81,109.63 13.75,109.63 v13.46,109.92
USIM_CLK  (via drill 0.3)
  Top 0.203: U1.16 2.27,52.2 v2.26,52.21 | v25.05,83.54 25.05,83.96 24.9,84.11 24.9,84.66 25.29,85.04 26.31,85.04 R7.2
  Route2 0.203: v2.26,52.21 3.5,50.98 3.5,49.59 4.17,48.91 10.15,48.91 13.26,52.03 13.26,67.72 22.58,77.04 22.58,82.03 24.24,83.69 24.9,83.69 v25.05,83.54
USIM_DATA  (via drill 0.3)
  Top 0.203: U1.15 3.73,53.46 v2.2,53.46 | v25.56,84.38 25.63,84.46 R8.2
  Route2 0.203: v2.2,53.46 3.88,51.78 3.88,49.75 4.33,49.3 9.99,49.3 12.91,52.22 12.91,67.86 22.23,77.18 22.23,82.17 24.43,84.38 v25.56,84.38
USIM_GND  (via drill 0.3)
  Top 0.203: U1.10 v2.42,60 v2.41,59.99 | 34.6,86.52 v35.02,86.94 | J1.C5 34.6,86.52 | 34.6,86.52
  Route2 0.203: v2.41,59.99 5.01,57.39 5.01,50.68 5.26,50.43 9.52,50.43 11.84,52.74 11.84,68.31 21.16,77.63 21.16,82.62 25.49,86.94 v35.02,86.94
  Bottom 0.203: v35.02,86.94 35.04,86.92 C46.2
USIM_PRE  (via drill 0.3)
  Top 0.203: U1.13 2.24,56.1 v2.22,56.12 | v25.45,85.95 26.07,85.95 26.44,85.95 26.46,85.95 R48.2
  Route2 0.203: v2.22,56.12 4.65,53.69 4.65,50.32 4.9,50.07 9.67,50.07 12.2,52.6 12.2,68.16 21.52,77.48 21.52,82.47 25,85.95 v25.45,85.95
USIM_RST  (via drill 0.3)
  Top 0.203: U1.17 2.42,50.9 v2.38,50.86 | R6.2 26.48,83.17 v26.27,82.96
  Route2 0.203: v2.38,50.86 3.11,50.13 3.11,49.43 4.01,48.53 10.31,48.53 13.62,51.84 13.62,67.57 22.94,76.89 22.94,81.88 23.79,82.74 26.04,82.74 v26.27,82.96
USIM_VDD  (via drill 0.3)
  Top 0.203: U1.14 2.21,54.8 v2.2,54.81 | D5.1 32.1,85.25 J1.C1 | J1.C1 | J1.C1 34.77,85.25 v34.98,85.04
  Route2 0.203: v2.2,54.81 4.27,52.74 4.27,49.91 4.49,49.69 9.83,49.69 12.55,52.41 12.55,68.01 21.87,77.33 21.87,82.32 24.59,85.04 v34.98,85.04
  Bottom 0.229: R9.1 36.88,81.58 37.04,81.75 37.04,84.7 36.64,85.1 35.04,85.1
  Bottom 0.508: C46.1 35.04,85.1 v34.98,85.04
V_BATT  (via drill 0.3, 0.41)
  Top 0.305: C40.2 C39.2 17.67,93.41 U4.1 | R49.1 5.24,104.16 4.3,104.16 3.5,103.36 D7.A D8.A 3.5,97.34 | D9.A 3.5,97.34 | 3.5,97.34 7.18,97.34 D11.A 8.12,96.4 v8.12,94.81
  Top 0.508: U5.1 17.37,87.51 C44.2 C45.2 15.59,87.32 v15.46,87.45 | U1.58 28.17,78.15 v28.68,78.66 | U1.59 26.87,78.47 v26.68,78.66 | C40.2 16.62,93.16 v15.46,93.16 | U1.60 25.57,78.45 v25.78,78.66 | U1.57 29.47,78.55 v29.58,78.66
  Route15 2.54: v25.78,78.66 v29.58,78.66 34.28,78.66 35.44,77.5 35.44,38.54 40.77,33.21 40.77,29.17 40.53,28.93 v37.7,28.93
  Bottom 0.305: v15.46,93.16 9.75,93.16 8.12,94.79 v8.12,94.81
  Bottom 0.508: U11.4 37.71,29.83 37.71,28.88 37.7,28.89 v37.7,28.93
  Bottom 1.27: S1.3 16.46,95.19 15.46,94.18 v15.46,93.16 v15.46,87.45
  Bottom 3.048: v25.78,78.66 26.02,78.42 37.47,78.42 38.87,79.82 38.87,93.91 37.59,95.19 S1.3
  other vias: 27.78,78.66 38.63,29.19 38.37,28.32 39.24,28.55
  pour Top (isolate 0.254, no thermals): 15.79,79.82 29.95,79.82 29.97,79.8 31.4,79.8 31.55,79.65 31.55,78.14 31.49,78.08 29.95,78.07 15.76,78.07 15.76,79.78
  pour Bottom (isolate 0.254, no thermals): 37.27,30.18 41.44,30.18 41.59,30.03 41.59,27.92 41.4,27.73 37.2,27.73 37.2,30.16 37.24,30.2
V_USB  (via drill 0.35)
  Top 0.261: J2.1 16.27,113.2 16.54,113.2 16.55,113.2
  Top 0.305: U1.71 11.19,76.53 11.19,80.82 11.81,81.44 11.81,101.3 11.14,101.97 11.13,101.97 | v10.51,101.35 11.13,101.97 | 11.13,101.97 8.33,101.97 7.5,101.14 D2.A
  Top 0.508: U3.4 21.17,105.11 20.9,105.38 20.9,107.42 21.06,107.58 21.06,110.52 20.07,111.51 18.37,111.51 D13.C | 16.46,113.1 17.82,111.74 D13.C | D13.C v17.82,110.29
  Route15 0.305: v10.51,101.35 11.99,102.83 13.62,102.83 15.81,105.02 15.81,106.21 17.82,108.22 v17.82,110.29
  pour Top (no thermals): 16.25,113.64 16.25,112.54 16.45,112.34 16.85,112.34 17.25,111.94 17.55,111.94 17.55,112.44 17.35,112.64 16.55,113.44 16.55,113.64
VDD3V3_FC20  (via drill 0.3)
  Bottom 0.203: R18.1 28.02,33.46 28.02,31.84 26.58,30.4 L1.2
  Bottom 1.27: v11.02,39.32 11.07,39.27 11.07,39.05
  Bottom 2.54: L1.2 17.11,39.05 11.07,39.05
  other vias: 11.02,38.4 10.31,38.9 11.75,38.9
  pour Top (isolate 0.254, no thermals): 10.56,35.31 7.43,35.31 7.43,35.37 7.34,35.37 7.34,41.91 8.66,41.91 8.67,41.92 12,41.92 12.2,41.72 12.2,37.51 12.21,37.5 11.13,37.62 11.1,37.59 8.79,37.59 8.63,37.43 8.67,36.21 9,35.88 10.5,35.88 10.58,35.8 10.58,35.34
  pour Bottom (isolate 0.254, no thermals): 27.82,31.32 27.82,24.82 27.62,24.62 26.34,24.62 25.9,25.06 25.9,31.54 27.63,31.54 27.81,31.36
VDD_1V8  (via drill 0.3, 0.35)
  Top 0.203: v21.18,88.26 20.98,88.06 20.98,87.51 | v21.18,88.26 21.44,88.52 R56.1 23.57,88.52 C43.2 C42.2 C41.2 | R55.2 18.88,89.06 19.68,88.26 v21.18,88.26
  Top 0.305: U5.5 20.98,87.51 | v33.2,101.92 35.35,101.92 36.64,100.63 43.36,100.63 v44.19,101.46
  Top 0.508: v33.2,101.92 27.96,101.92 26.71,103.17 21.83,103.17 20.86,102.2 v20.86,101.74
  Route15 0.203: v44.19,101.46 44.19,103.97 v44.88,104.66 44,105.54 42.62,105.54 40.81,107.36 40.81,109.64 38.26,112.18 v38.26,113.19
  Route15 0.508: v21.18,88.26 21.18,88.82 20.57,89.43 20.57,90.1 20.86,90.39 v20.86,101.74
  Bottom 0.203: U7.29 39.53,109.54 39.33,109.74 C65.2 C66.2 38.23,110.41 R63.2 | R71.1 44.83,104.62 v44.88,104.66 | R72.1 43.38,101.16 43.69,101.46 v44.19,101.46 | v38.26,113.19 37.33,112.26 R63.2 | R64.2 37.33,112.1 R63.2
  Bottom 0.508: R74.1 33.77,101.92 v33.2,101.92
VDD_3.3V  (via drill 0.3, 0.35)
  Top 0.203: v24.4,92.4 28.76,92.4 33.9,97.54 35.26,97.54 37.82,100.1 v44.05,100.1
  Top 0.305: C36.2 C37.2 C38.2 23.62,92.08 | U4.5 22.43,93.41 22.68,93.16 R53.1 23.38,92.32 23.62,92.08 | 23.62,92.08 24.08,92.08 v24.4,92.4
  Route15 0.203: v44.05,100.1 44.05,100.36 45.85,102.15 45.85,106.37 44.84,107.37 44.4,107.37 v44.3,107.47 44.01,107.76 v44.01,110.11
  Bottom 0.203: R73.1 v44,110.11 v44.01,110.11 | R65.2 44.3,107.82 v44.3,107.47
VDD_EXT  (via drill 0.3, 0.35, 0.41)
  Top 0.203: v31.36,26.48 30.99,26.85 29.25,26.85 28.45,27.65 28.45,27.92 | v26.37,39.5 27.45,38.42 C16.2 | R40.2 28.62,33.76 28.71,33.85 29.26,33.85 29.65,33.47 29.65,28.59 28.98,27.92 28.45,27.92 | R30.2 28.45,27.92
  Top 0.305: C13.2 C14.2 C15.2 C16.2 | v7.72,21.55 8.56,21.55 R2.1 | v32.51,89.68 33.1,89.68 R47.1 | R59.1 15.34,85.46 15.01,85.13 15.01,83.55 15.28,83.28 v16.48,83.28
  Top 0.508: U2.11 v26.35,35.62 27.41,35.62 C13.2 | U1.7 2.64,67 v2.61,66.97
  Route2 0.305: v16.48,83.28 21.25,83.28 25.32,87.35 28.43,87.35 30.76,89.68 v32.51,89.68 | v16.28,11.76 16.4,11.88 19.62,11.88 v19.62,11.8
  Route2 0.508: v3.21,83.44 2.02,83.44 1.38,82.8 1.38,66.96 | v6.45,27.81 8.24,27.81 10.58,25.47 10.58,22.68 9.45,21.55 v7.72,21.55 | v2.61,66.97 v2.6,66.96 1.38,66.96 | 1.38,66.96 1.38,49.81 3.48,47.71 4.37,47.71 5.7,46.38 5.7,35.73 v6.39,35.04 9.33,35.04 10,35.71 10,35.72 26.25,35.72 v26.35,35.62
  Route15 0.203: v26.37,39.5 27.16,39.5 29.75,36.91 29.75,35.97 31.95,33.78 31.95,27.07 v31.36,26.48
  Route15 0.305: v7.72,21.55 7.72,13.45 9.47,11.7 16.22,11.7 v16.28,11.76
  Route15 0.508: v3.21,83.44 16.32,83.44 v16.48,83.28 | v6.39,35.04 6.39,33.75 v6.26,33.62 6.26,32.24 v6.21,32.19 6.49,31.91 6.49,30.3 6.44,30.25 v6.44,30.03 v6.45,30.02 v6.45,27.81
  Bottom 0.152: 6.51,27.78 6.5,27.77 6.49,27.77 v6.45,27.81 | v6.45,30.02 v6.44,30.03 | R22.2 6.22,32.2 v6.21,32.19 | R21.2 v6.26,33.62 | R20.2 v6.39,35.04
  Bottom 0.203: C23.1 R43.1 15.19,11.66 R44.1 | R83.2 R26.2 23.92,13.86 23.02,12.96 20.78,12.96 v19.62,11.8
  Bottom 0.293: 6.51,27.78 R24.2 | R23.2 v6.45,30.02 | v6.39,35.04
  Bottom 0.305: v16.28,11.76 R44.1 | R19.2 R20.2 | R82.1 19.62,17.86 v19.62,11.8 19.62,9.72 20.68,8.66 27.64,8.66 C81.1 28.2,10.32 U6.1
VDD_MCU  (via drill 0.35)
  Route15 0.305: v6.98,16.84 7.26,16.57 7.26,13.26 10.26,10.26 19.9,10.26 22.98,7.19 34.28,7.19 37.06,9.96 37.08,9.96 v37.08,10.16
  Bottom 0.305: WIPHONE_DAUGHTERBOARD-FOOTPRINT1.14 6.67,16.84 v6.98,16.84 | U6.14 35.79,10.57 C27.1 36.2,10.16 v37.08,10.16
W_DISABLE_EC25  (via drill 0.3)
  Top 0.203: U1.4 v2.29,70.9
  Route2 0.203: v2.41,22.65 3.1,22.65 3.23,22.78 5.1,22.78 8.94,18.94 v13.78,18.94
  Bottom 0.203: v13.78,18.94 13.78,16.96 12.98,16.16 10.77,16.16 C22.1 12.07,15.48 Q4.3 | v2.29,70.9 4.97,70.9 5.62,70.25 5.62,61.64 4.8,60.82 4.8,51.69 6.22,50.27 6.22,43.23 1.86,38.88 1.86,23.13 2.34,22.65 v2.41,22.65
W_DISABLE_MCU  (via drill 0.35)
  Route2 0.203: v13.15,12.94 13.15,5.44 13.63,4.96 v14.05,4.96
  Bottom 0.203: v13.15,12.94 13.15,14.04 13.13,14.06 13.13,14.09 Q4.1 | R92.2 38.88,8.55 38.88,7.01 36.83,4.96 v14.05,4.96
WAKE_ON_WIRELESS  (via drill 0.3)
  Top 0.203: R1.1 R2.2 7.88,22.41 7.48,22.81 v7.5,22.84 | U1.135 5.92,60.6 v5.92,60.51
  Route15 0.203: v5.92,60.51 3.04,57.63 3.04,49.92 0.77,47.65 0.77,36.77 1.23,36.31 1.23,24.76 2.48,23.51 3.16,22.84 v7.5,22.84
WAKEUP_IN_EC25  (via drill 0.3, 0.41)
  Top 0.203: U1.1 v2.27,74.8
  Route2 0.203: v4.85,22 4.85,21.11 9.49,16.46 v14.58,16.46
  Bottom 0.203: v14.58,16.46 14.78,16.26 C21.1 16.87,15.48 Q3.3 | v2.27,74.8 6.33,70.74 6.33,61.03 7.22,60.14 7.22,42.99 2.58,38.35 2.58,24.27 v4.85,22
WAKEUP_IN_MCU  (via drill 0.35)
  Route2 0.203: v23.15,6.14 22.16,6.14 21.67,5.66 19.57,5.66 19.17,6.06 19.17,9.38 v17.55,11 | v38.2,7.29 38.2,12.48 v37.37,13.31
  Bottom 0.203: v17.55,11 17.93,11.38 17.93,14.09 Q3.1 | v23.15,6.14 36.95,6.14 38.15,7.34 v38.2,7.29 | v37.37,13.31 37.41,13.34 R91.2
WLAN_EN  (via drill 0.3)
  Top 0.203: U1.136 5.88,58.56 v5.88,58.46 | v22.15,31.26 22.15,33.25 22.32,33.42 U2.9 27.02,33.42 C18.1 R40.1
  Route2 0.203: v2.15,40.19 4.2,38.13 4.2,29.48 5.03,28.64 8.13,28.64 9.91,26.86 21.23,26.86 23.11,28.74 23.11,30.08 22.1,31.09 22.1,31.26 v22.15,31.26
  Route15 0.203: v5.88,58.46 3.4,55.98 3.4,49.78 1.22,47.6 1.22,41.11 v2.15,40.19
WLAN_SLP_CLK  (via drill 0.3)
  Top 0.203: U1.118 9.27,71.95 v9.27,71.99 | v14.36,42.84 14.46,42.74 R25.1
  Route2 0.203: v14.36,42.84 14.36,67.71 15.72,69.07 15.91,69.07 v15.98,69
  Bottom 0.203: v15.98,69 12.26,69 v9.27,71.99

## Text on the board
bPlace: v1.1
tNames: J2
_tNames: C86 | C85 | J3 | D6 | D22 | C40 | C39 | U4 | C88 | D4 | R53 | C87 | C38 | R51 | R55 | R54 | C37 | Q10 | C36 | U3 | R56 | C43 | R50 | C45 | C44 | C42 | C89 | D2 | R57 | C41 | C90 | C26 | FL1 | R59 | R58 | D3 | U5 | L2 | C68 | C69 | ANT1 | C83 | L5 | U1 | C74 | C75 | ANT4 | L3 | C70 | C71 | ANT2 | D7 | R32 | R34 | R36 | R38 | R79 | R1 | R2 | D8 | R11 | C72 | L4 | C73 | D9 | R78 | ANT3 | J1 | R3 | R24 | U2 | R4 | R23 | C1 | R5 | R22 | R12 | R21 | R13 | R20 | R14 | R19 | S1 | J11 | R83
_bNames: C79 | C80 | R64 | C66 | C65 | C81 | C61 | C55 | R70 | R75 | C76 | R10 | R60 | C52 | R63 | C60 | R66 | R73 | C78 | C77 | R67 | C59 | R65 | R76 | C54 | R69 | R68 | C67 | C31 | C35 | R77 | R62 | U7 | D1 | C28 | C29 | C30 | C32 | C33 | C34 | C50 | C58 | C53 | C48 | R61 | R71 | C47 | C49 | C57 | C4 | C8 | C56 | R74 | C51 | C62 | C63 | C64 | R72 | R40 | R39 | C6 | C2 | R80 | C46 | C3 | R7 | R8 | C5 | R29 | R28 | R27 | C18 | C19 | C10 | C7 | R6 | R9 | R30 | C16 | C15 | C14 | C13 | C17 | R25 | C11 | C12 | D5 | C9 | R15 | R18 | R16 | U6 | R17 | R49 | Q9 | C27 | L1 | C82 | R52 | Q8 | Q12 | Q11 | R82 | D10 | R81 | C20 | R42 | R48 | R46 | Q2 | Q1 | C22 | C21 | Q7 | C24 | R45 | R47 | R41 | Q5 | Q4 | Q3 | C25 | R31 | R26 | R44 | R33 | R37 | R43 | R35 | Q6 | C23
